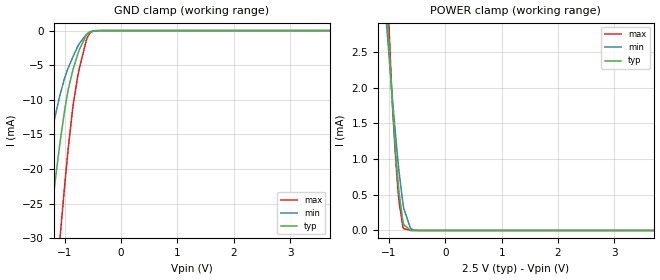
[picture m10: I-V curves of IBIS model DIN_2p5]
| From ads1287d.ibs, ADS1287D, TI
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|   Model
[Model]   DIN_2p5
Model_type   Input
Vinl = 0.75
Vinh = 1.75
|   typ   min   max
C_comp   2.259pF   1.924pF   2.539pF
[Voltage Range]   2.5   2.2   2.8
[Temperature Range]   27   125   -40
[Power Clamp Reference]   2.5   2.2   2.8
[GND Clamp Reference]   0   0   0
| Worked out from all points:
|   GND clamp passes 1 mA (typ) near -0.64 V on its own axis
|   POWER clamp passes 1 mA (typ) near -0.87 V on its own axis
[GND Clamp]
|   Voltage   I(typ)   I(min)   I(max)
-2.5V     -136.1mA   -88.5mA    -181.5mA
-1.532V   -49.29mA   -28.94mA   -76mA
-1.353V   -34.92mA   -20.1mA    -56.91mA
-1.248V   -27.11mA   -15.47mA   -46.06mA
-1.075V   -15.63mA   -8.997mA   -29.07mA
-962.5mV  -9.573mA   -5.883mA   -19mA
-850mV    -5.526mA   -3.695mA   -10.65mA
-745mV    -2.811mA   -1.907mA   -5.573mA
-617.5mV  -624.2uA   -552.4uA   -1.392mA
-550mV    -166.2uA   -241.1uA   -357.5uA
-392.5mV  -2.502uA   -19.12uA   -2.534uA
5V        0A         0A         0A
[POWER Clamp]
|   Voltage   I(typ)   I(min)   I(max)
-2.5V     32.31mA    25.39mA    39.43mA
-1.038V   3.118mA    2.832mA    3.592mA
-1.03V    3.005mA    2.754mA    3.437mA
-962.5mV  2.068mA    2.075mA    2.155mA
-932.5mV  1.693mA    1.787mA    1.674mA
-880mV    1.093mA    1.307mA    985.3uA
-842.5mV  716.5uA    990.3uA    590.9uA
-820mV    520.3uA    814.2uA    392.7uA
-737.5mV  80.72uA    306.8uA    26.65uA
-617.5mV  1.215uA    30.69uA    123nA
-512.5mV  3.553nA    1.842uA    0A
5V        0A         0A         0A
